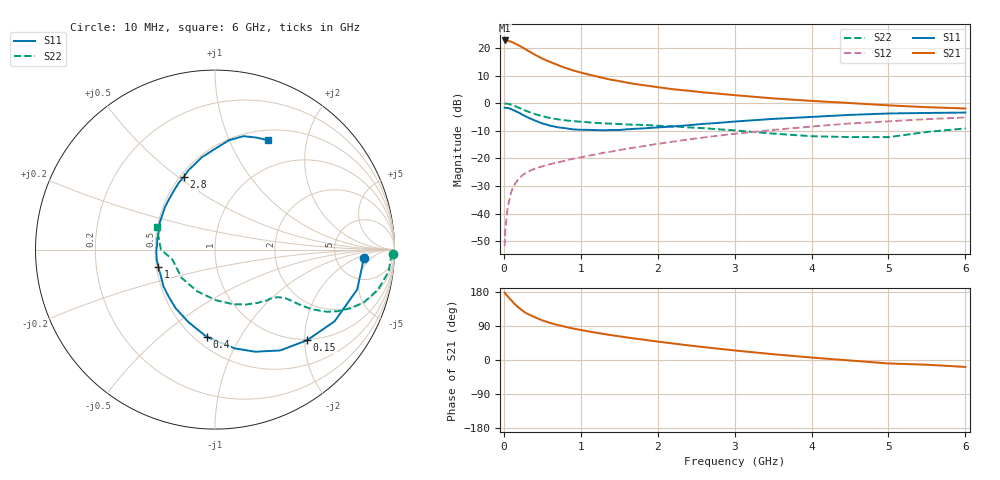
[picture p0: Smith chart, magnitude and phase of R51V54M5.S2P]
! SIEMENS Small Signal Semiconductors
! BFR183
! Si NPN RF Bipolar Junction Transistor in SOT23
! VCE = 1.5 V  IC = 4.5 mA
! Common Emitter S-Parameters:  May  1996
# GHz  S  MA  R  50
!  f  S11  S21  S12  S22
! GHz  MAG  ANG  MAG  ANG  MAG  ANG  MAG  ANG
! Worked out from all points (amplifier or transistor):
!   36 points, 10 MHz to 6 GHz, reference 50 ohm
!   highest |S21| = 22.7 dB at 10 MHz (marker M1)
!   |S21| within 3 dB of that: start of sweep to 271.1 MHz
!   unconditionally stable (mu >= 1): 1.069 GHz to 2.726 GHz
!   at 250 MHz: K = 0.40, MSG = 23.0 dB, |S12| = -25.9 dB
!   at 1.4 GHz: K = 1.07, MAG = 11.4 dB, |S12| = -17.5 dB
!   at 6 GHz: K = 0.91, MSG = 1.6 dB, |S12| = -5.2 dB
!   S11 on the Smith chart (normalised r, x): 10 MHz: 10, -3; 150 MHz: 0.98, -2.05; 400 MHz: 0.57, -0.73; 1 GHz: 0.51, -0.11; 2.8 GHz: 0.52, +0.53; 6 GHz: 0.62, +1.40
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0.01  0.8305 -3.2  13.62 177.9  0.0026 88.5  0.9906 -1.4
0.02  0.8251 -6.5  13.6 175.0  0.0052 86.5  0.9807 -2.9
0.05  0.8227 -15.7  13.4 168.0  0.0133 81.7  0.9754 -7.2
0.1  0.777 -30.9  12.87 156.7  0.0258 73.8  0.935 -13.8
0.15  0.7201 -44.5  11.89 145.8  0.0359 68.0  0.8803 -19.5
0.2  0.6692 -57.1  10.98 137.1  0.044 63.7  0.8236 -23.4
0.25  0.6115 -68.5  10.04 129.0  0.0508 59.5  0.7641 -26.7
0.3  0.5615 -78.7  9.114 122.6  0.0564 57.2  0.7146 -29.0
0.4  0.4885 -95.4  7.581 113.1  0.0654 54.0  0.6386 -31.5
0.5  0.4304 -110.1  6.398 104.6  0.0722 52.9  0.5811 -32.7
0.6  0.3935 -123.9  5.575 97.9  0.0787 52.8  0.5397 -33.4
0.7  0.3671 -135.0  4.907 92.4  0.0849 53.1  0.5114 -33.8
0.8  0.3529 -144.6  4.344 87.6  0.0917 53.4  0.4894 -34.3
1  0.3304 -162.7  3.578 79.2  0.105 54.3  0.4622 -35.3
1.1  0.3295 -171.0  3.3 75.5  0.1122 54.9  0.4513 -36.2
1.6  0.3371 157.9  2.354 59.5  0.1501 56.2  0.4121 -41.5
2.2  0.3792 132.7  1.788 43.6  0.2018 54.7  0.381 -51.3
2.8  0.4415 113.1  1.483 29.6  0.2599 50.5  0.3363 -65.1
3.5  0.5201 98.0  1.222 15.3  0.3281 43.1  0.2821 -88.9
4.5  0.6144 82.7  1.006 -1.3  0.4303 30.8  0.2438 -139.4
5.5  0.6658 69.6  0.847 -12.5  0.5142 18.1  0.3019 179.7
6  0.677 64.3  0.803 -18.3  0.5518 10.0  0.3495 158.5
